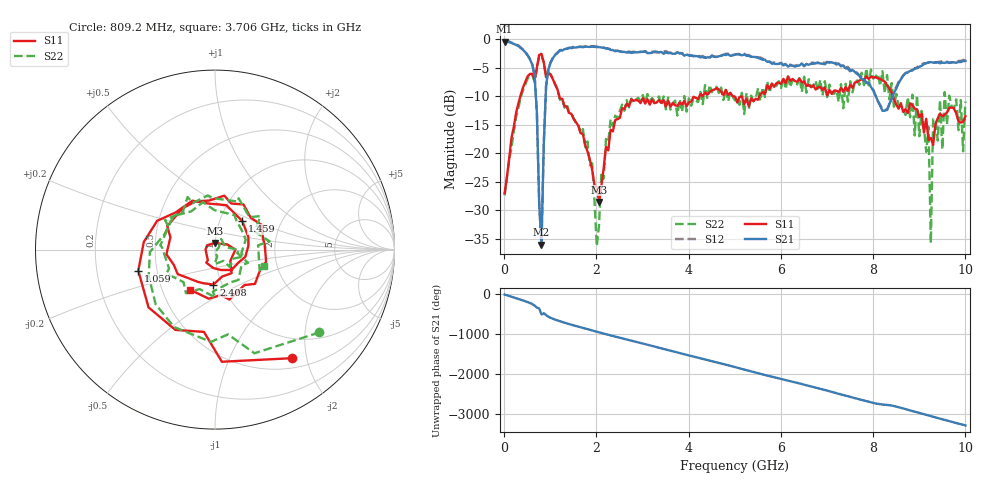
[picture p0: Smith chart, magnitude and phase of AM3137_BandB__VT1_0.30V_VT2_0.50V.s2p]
! Date/Time: Tue, Nov 13, 2018 4:51 PM
! Network Analyzer: Agilent Technologies E8364B Rev: A.07.50.67
! Sweep from 0.010 to 10.000 GHz, 201 Points, Sweep Type: LIN
! Power Supply: 0.300 V, -0.000 A
# Hz S DB R 50
!freq MagS11 AngS11 MagS21 AngS21 MagS12 AngS12 MagS22 AngS22
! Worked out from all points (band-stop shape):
!   201 points, 10 MHz to 10 GHz, reference 50 ohm
!   highest |S21| = -0.42 dB at 10 MHz (marker M1); lowest = -36.1 dB at 809.2 MHz (marker M2)
!   |S21| within 3 dB of the highest: start of sweep to 550.2 MHz; 1.051 GHz to 5.552 GHz (4.501 GHz wide, 136 % of centre)
!   lowest |S11| = -28.6 dB at 2.058 GHz (marker M3), VSWR 1.08, Z = 49.8 + j3.72 ohm
!   |S11| at or under -10 dB: 1.195 GHz to 4.234 GHz (3.039 GHz wide, 112 % of centre); 4.953 GHz to 5.536 GHz (582.4 MHz wide, 11.1 % of centre); 8.428 GHz to end of sweep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
!   |S22| runs from -36.3 to -2.6 dB; largest |S21 - S12| = 0.036
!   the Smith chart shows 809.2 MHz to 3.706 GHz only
!   S11 on the Smith chart (normalised r, x): 809.2 MHz: 0.65, -1.75; 1.059 GHz: 0.39, -0.11; 1.459 GHz: 1.28, +0.43; 2.408 GHz: 0.91, -0.37; 3.706 GHz: 0.69, -0.33
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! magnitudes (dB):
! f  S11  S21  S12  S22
! 10 MHz  -27.0  -0.4  -0.2  -27.4
! 309.7 MHz  -11.2  -1.2  -1.1  -12.0
! 659.4 MHz  -7.1  -6.3  -6.2  -7.5
! 809.2 MHz  -2.6  -36.1  -36.2  -2.6
! 909.1 MHz  -6.7  -8.2  -8.2  -6.4
! 1.059 GHz  -7.1  -3.3  -3.2  -6.9
! 1.459 GHz  -13.1  -1.6  -1.5  -13.1
! 1.708 GHz  -16.7  -1.4  -1.3  -15.8
! 2.058 GHz  -28.6  -1.4  -1.3  -32.6
! 2.208 GHz  -18.9  -1.6  -1.6  -17.5
! 2.408 GHz  -14.2  -2.1  -2.0  -13.4
! 3.357 GHz  -10.7  -2.3  -2.3  -10.0
! 3.706 GHz  -11.6  -2.5  -2.5  -10.8
! 5.005 GHz  -10.1  -2.7  -2.7  -10.7
! 6.703 GHz  -8.1  -4.3  -4.1  -8.2
! 8.352 GHz  -8.6  -11.3  -11.4  -10.6
! 9.201 GHz  -17.7  -4.1  -4.1  -15.4
! 9.251 GHz  -17.3  -4.0  -4.0  -35.8
! 9.301 GHz  -18.6  -4.1  -4.1  -14.0
! 9.9 GHz  -14.6  -4.0  -3.8  -10.7
! 9.95 GHz  -14.5  -3.8  -3.6  -19.7
! 10 GHz  -13.5  -3.8  -3.7  -10.9
